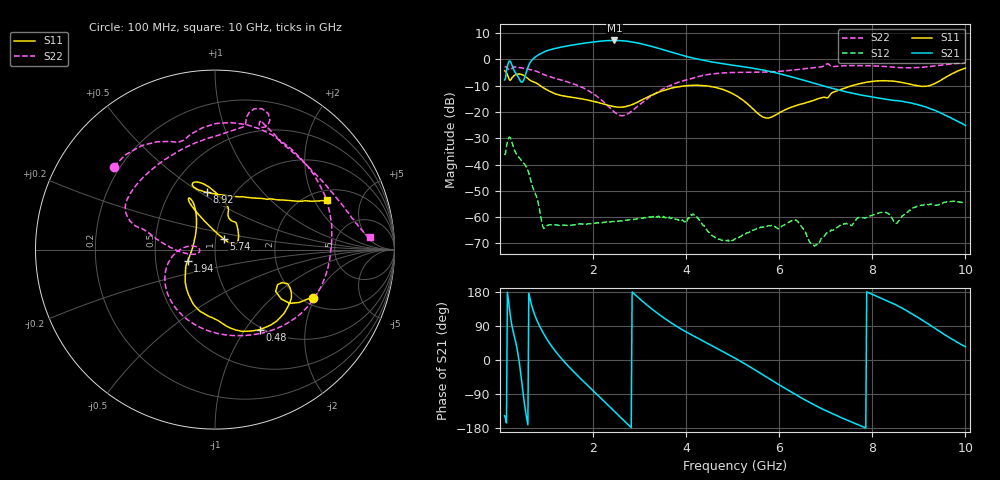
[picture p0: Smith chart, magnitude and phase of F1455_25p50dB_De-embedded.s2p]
! Integrated Device Technology
! Corporate Headquarters
! 6024 Silver Creek Valley Road
! San Jose, CA 95138  USA
! Phone:  1-408-284-8200
! Toll Free:  1-800-223-1366
! Webpage:  http://www.idt.com/
! Timing and RF Division
! 515 Groton Road, Suite 102
! Westford, MA 01886-6024
! Device:  F1455
! Description: 6-bit 0.5 dB Transmit Variable Gain Amplifier
! Frequency:  1400.0 -  2300.00 MHz
! Package:  6x6 mm Thin QFN Plastic Package: 28 pin
! State:  51
! Atten State:  25.5 dB
! Voltage:  +5.00 Volts
! Current:  217.607 mA
! Data:  The device was measured on a the F1455 evaluation board which has
!  individual transmission lines to the RF pins.  Data was collected
!  using a calibrated network analyzer.  The evaluation board was
!  de-embedded using a TRL calibration technique.
!  The reference plane is the edge of the package pin.
!  Pin  1 = CSb
!  Pin  2 = DATA
!  Pin  3 = CLK
!  Pin  4 = RSET
!  Pin  5 = GND
!  Pin  6 = RFIN  = Port 1
!  Pin  7 = GND
!  Pin  8 = NC
!  Pin  9 = NC
!  Pin 10 = NC
!  Pin 11 = NC
!  Pin 12 = NC
!  Pin 13 = NC
!  Pin 14 = /STBY
!  Pin 15 = GND
!  Pin 16 = RFOUT  = Port 2
!  Pin 17 = GND
!  Pin 18 = NC
!  Pin 19 = NC
!  Pin 20 = NC
!  Pin 21 = GND
!  Pin 22 = NC
!  Pin 23 = GND
!  Pin 24 = NC
!  Pin 25 = NC
!  Pin 26 = NC
!  Pin 27 = GND
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# GHz S dB R 50
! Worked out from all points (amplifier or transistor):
!   496 points, 100 MHz to 10 GHz, reference 50 ohm
!   highest |S21| = 7.2 dB at 2.46 GHz (marker M1)
!   |S21| within 3 dB of that: 1.194 GHz to 3.407 GHz (2.212 GHz wide, 96.2 % of centre)
!   unconditionally stable (mu >= 1): start of sweep to end of sweep
!   at 1.74 GHz: K = 299.30, MAG = 6.5 dB, |S12| = -62.6 dB
!   at 5.06 GHz: K = 1098.76, MAG = -0.5 dB, |S12| = -68.2 dB
!   at 10 GHz: K = 636.92, MAG = -16.4 dB, |S12| = -54.4 dB
!   S11 on the Smith chart (normalised r, x): 100 MHz: 2.27, -1.94; 480 MHz: 0.97, -1.18; 1.94 GHz: 0.73, -0.09; 5.74 GHz: 1.09, +0.13; 8.92 GHz: 0.75, +0.54; 10 GHz: 2.45, +2.54
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0.1  -4.30 -26.1  -7.82 -147.1  -36.37 47.6  -2.75 140.7
0.18  -6.73 -36.7  -1.30 160.7  -30.15 -6.6  -3.71 112.5
0.26  -6.97 -25.2  -2.32 88.6  -31.68 -77.2  -3.33 96.0
0.38  -5.62 -42.5  -6.33 21.4  -36.68 -118.1  -3.01 58.1
0.48  -5.82 -60.5  -8.70 -69.9  -38.82 -149.8  -3.27 31.8
0.66  -8.09 -87.9  -0.86 154.3  -45.94 141.1  -3.92 -9.9
0.8  -9.21 -105.8  1.40 102.9  -53.00 111.1  -4.64 -41.0
0.96  -11.10 -123.6  2.93 65.0  -64.12 129.6  -5.89 -70.5
1.34  -13.79 -143.7  4.76 1.1  -63.11 112.9  -7.98 -121.0
1.76  -15.00 -153.4  6.03 -52.4  -62.59 82.9  -10.60 -157.9
1.94  -15.69 -157.6  6.48 -73.8  -62.52 75.8  -12.31 -170.6
2.2  -16.85 -166.9  7.00 -104.5  -62.12 65.7  -15.72 174.7
2.46  -18.02 176.1  7.20 -135.6  -61.66 56.8  -20.04 172.3
2.84  -17.19 141.7  6.62 179.4  -60.96 46.9  -19.56 -167.0
3.4  -12.55 117.0  4.23 121.8  -59.59 27.9  -12.31 177.7
4.1  -9.87 116.4  0.70 67.3  -59.10 9.5  -7.39 164.0
5.06  -13.62 114.5  -2.36 4.1  -68.20 28.0  -4.96 148.8
5.74  -22.32 51.5  -4.34 -45.8  -63.51 24.4  -4.84 120.5
6.7  -15.83 36.9  -8.83 -115.2  -70.47 -141.6  -3.24 78.8
8.36  -8.17 108.6  -15.35 153.5  -58.88 67.9  -2.82 62.8
8.92  -9.84 97.8  -16.96 116.7  -56.21 88.7  -3.15 40.4
10  -3.32 23.9  -25.12 35.1  -54.38 17.4  -1.26 4.7
